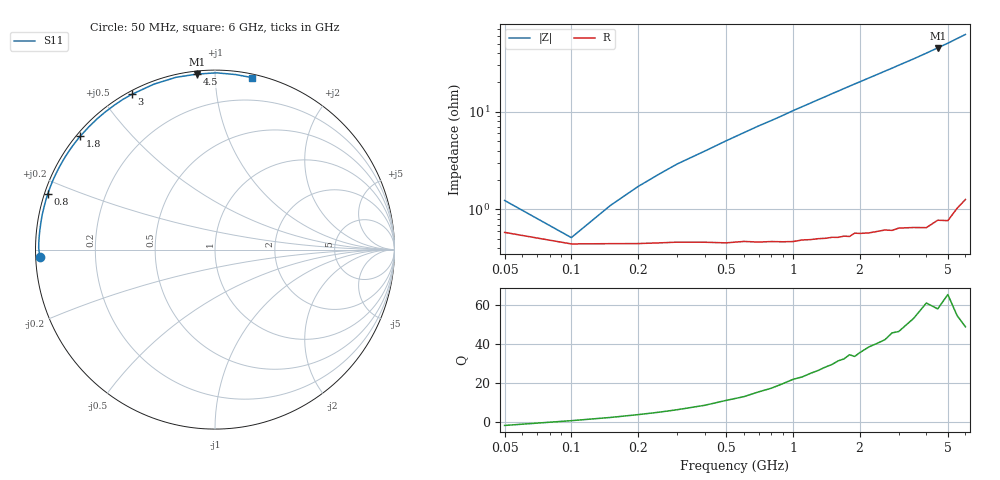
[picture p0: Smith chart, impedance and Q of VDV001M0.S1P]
! Infineon Technologies  Discrete & RF Semiconductors
! BBY 55-03
! Si Tuning Diode in SOD323
! VR =
! S-Parameters:  June  1999
# GHz  S  MA  R  50
!  f  S11
! GHz  MAG  ANG
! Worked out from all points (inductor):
!   34 points, 50 MHz to 6 GHz, reference 50 ohm
!   read as one part to ground: L = 1.45 nH near 200 MHz
!   highest Q = 61.2 at 4.5 GHz (marker M1), where L = 1.6 nH
!   S11 on the Smith chart (normalised r, x): 50 MHz: 0.01, -0.02; 800 MHz: 0.01, +0.16; 1.8 GHz: 0.01, +0.37; 3 GHz: 0.01, +0.60; 4.5 GHz: 0.02, +0.90; 6 GHz: 0.03, +1.24
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0.05  0.977 -177.5
0.1  0.9824 179.4
0.15  0.9823 177.7
0.2  0.9823 176.2
0.3  0.9817 173.4
0.5  0.9821 168.5
0.7  0.982 163.7
0.8  0.9819 161.5
0.9  0.9821 159.2
1  0.9821 156.8
1.2  0.9816 152.4
1.3  0.9814 150.2
1.4  0.9814 148.1
1.5  0.9812 145.9
1.6  0.9814 143.9
1.8  0.9815 139.8
2  0.9807 135.9
2.2  0.9809 132.1
2.4  0.9808 128.5
2.6  0.9808 124.9
2.8  0.9816 121.5
3  0.9812 118.1
3.5  0.9825 110.3
4  0.9842 102.8
4.5  0.983 95.8
5  0.9849 89.5
5.5  0.982 83.3
6  0.9802 77.8
